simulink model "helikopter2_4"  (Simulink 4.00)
settings: Solver=ode1  SolverMode=SingleTasking  StartTime=0.0  StopTime=999999  FixedStep=0.005  MaxStep=10  RelTol=1e-3  AbsTol=1e-3
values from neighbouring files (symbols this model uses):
  a = [0 0 0;0 0 1;0 0 0]    [init3.m]
  b = [k3 k3;0 0;k1 -k1]    [init3.m]
  c = [ 1 0 0 0 0 0    [init3.m]
  L = (place(a',c',p))'    [init3.m]
undefined symbols (not defined in the file or in its folder): simget
libraries: qctools x7

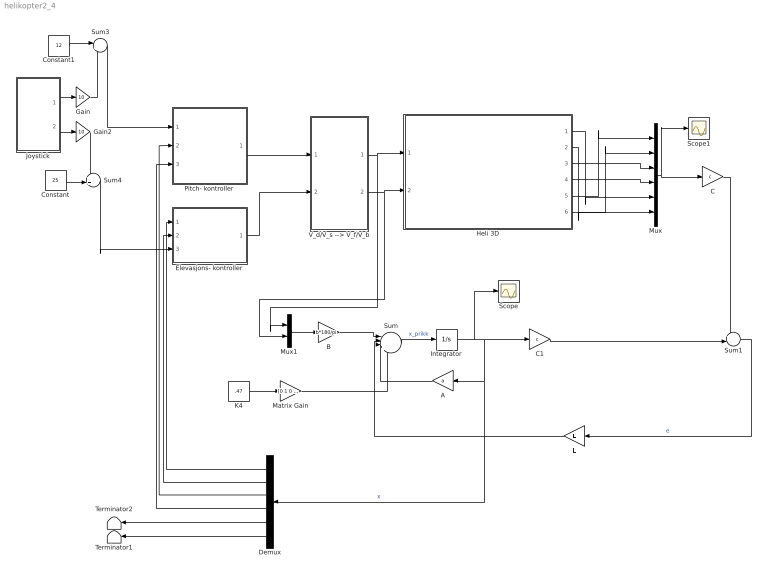
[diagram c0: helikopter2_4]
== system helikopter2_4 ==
  A : Gain  Orientation=left  Gain=a  Multiplication=Matrix(K*u)  SaturateOnIntegerOverflow=on
  B : Gain  Gain=b*180/pi  Multiplication=Matrix(K*u)  SaturateOnIntegerOverflow=on
  C : Gain  Gain=c  Multiplication=Matrix(K*u)  SaturateOnIntegerOverflow=on
  C1 : Gain  Gain=c  Multiplication=Matrix(K*u)  SaturateOnIntegerOverflow=on
  Constant : Constant  Value=25
  Constant1 : Constant  Value=12
  Demux : Demux  Orientation=left  Outputs=6  BusSelectionMode=off
  Elevasjons- kontroller : Subsystem
  Gain : Gain  Gain=10  Multiplication=Element-wise(K.*u)  SaturateOnIntegerOverflow=on
  Gain2 : Gain  Gain=10  Multiplication=Element-wise(K.*u)  SaturateOnIntegerOverflow=on
  Heli 3D : Subsystem
  Integrator : Integrator  ExternalReset=none  InitialConditionSource=internal  InitialCondition=0  LimitOutput=off  UpperSaturationLimit=inf  LowerSaturationLimit=-inf  ShowSaturationPort=off  ShowStatePort=off  AbsoluteTolerance=auto
  Joystick : Subsystem
  K4 : Constant  Value=.47
  L : Gain  Orientation=left  Gain=L  Multiplication=Matrix(K*u)  SaturateOnIntegerOverflow=on
  Matrix Gain : Gain  Gain=[0 1 0 0 0 0]'  Multiplication=Matrix(K*u)  SaturateOnIntegerOverflow=on
  Mux : Mux  Inputs=6
  Mux1 : Mux  Inputs=2
  Pitch- kontroller : Subsystem
  Scope : Scope
  Scope1 : Scope
  Sum : Sum  Inputs=|++++  SaturateOnIntegerOverflow=on
  Sum1 : Sum  Inputs=+-|  SaturateOnIntegerOverflow=on
  Sum3 : Sum  Inputs=|++  SaturateOnIntegerOverflow=on
  Sum4 : Sum  Inputs=++|  SaturateOnIntegerOverflow=on
  Terminator1 : Terminator
  Terminator2 : Terminator
  V_d/V_s --> V_f/V_b : Subsystem
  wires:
  V_d/V_s --> V_f/V_b/2(V_b) -> Heli 3D/2("V_b, motor bak"), Mux1/2
  V_d/V_s --> V_f/V_b/1(V_f) -> Heli 3D/1("V_f, motor foran"), Mux1/1
  Pitch- kontroller/1(V_d) -> V_d/V_s --> V_f/V_b/1(V_d)
  Elevasjons- kontroller/1(V_s) -> V_d/V_s --> V_f/V_b/2(V_s)
  Joystick/1(X Volt) -> Gain/1
  Joystick/2(Y Volt) -> Gain2/1
  Heli 3D/5("Elevasjon, (grader)") -> Mux/1
  Heli 3D/6(Elevasjonsrate (grader/sek)) -> Mux/2
  Heli 3D/3("Pitch, (grader)") -> Mux/3
  Heli 3D/4("Pitchrate, (grader/sek)") -> Mux/4
  Heli 3D/1("Vandring, (grader)") -> Mux/5
  Heli 3D/2("Vandringsrate, (grader/sek)") -> Mux/6
  Gain/1 -> Sum3/2
  B/1 -> Sum/1
  Sum/1 -> Integrator/1  "x_prikk"
  Mux/1 -> C/1, Scope1/1
  Integrator/1 -> C1/1, A/1, Demux/1, Scope/1  "x"
  C1/1 -> Sum1/2
  C/1 -> Sum1/1
  Sum1/1 -> L/1  "e"
  A/1 -> Sum/3
  L/1 -> Sum/2
  Demux/1 -> Elevasjons- kontroller/1("e, grader")
  Demux/2 -> Elevasjons- kontroller/2("e_dot, grader/sek")
  Demux/3 -> Pitch- kontroller/2("p, grader")
  Demux/4 -> Pitch- kontroller/3("p_dot, grader/sek")
  Demux/6 -> Terminator1/1
  Demux/5 -> Terminator2/1
  Constant1/1 -> Sum3/1
  Sum3/1 -> Pitch- kontroller/1("p_c, grader")
  Constant/1 -> Sum4/2
  Gain2/1 -> Sum4/1
  Sum4/1 -> Elevasjons- kontroller/3("e_c, grader")
  Mux1/1 -> B/1
  Matrix Gain/1 -> Sum/4
  K4/1 -> Matrix Gain/1

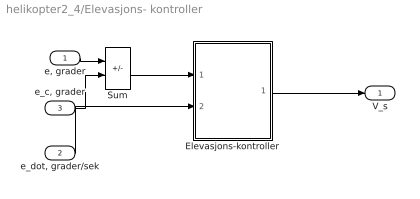
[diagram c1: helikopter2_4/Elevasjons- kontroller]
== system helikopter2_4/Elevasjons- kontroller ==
  "e, grader" : Inport  Port=1  LatchInput=off
  "e_dot, grader/sek" : Inport  Port=2  LatchInput=off
  "e_c, grader" : Inport  Port=3  LatchInput=off
  Elevasjons-kontroller : Subsystem
  Sum : Sum  Inputs=-+  SaturateOnIntegerOverflow=on
  V_s : Outport  Port=1  InitialOutput=0
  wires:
  Sum/1 -> Elevasjons-kontroller/1("e, grader")
  Elevasjons-kontroller/1(out_1) -> V_s/1
  "e, grader"/1 -> Sum/1
  "e_dot, grader/sek"/1 -> Elevasjons-kontroller/2("e, grader/sek")
  "e_c, grader"/1 -> Sum/2

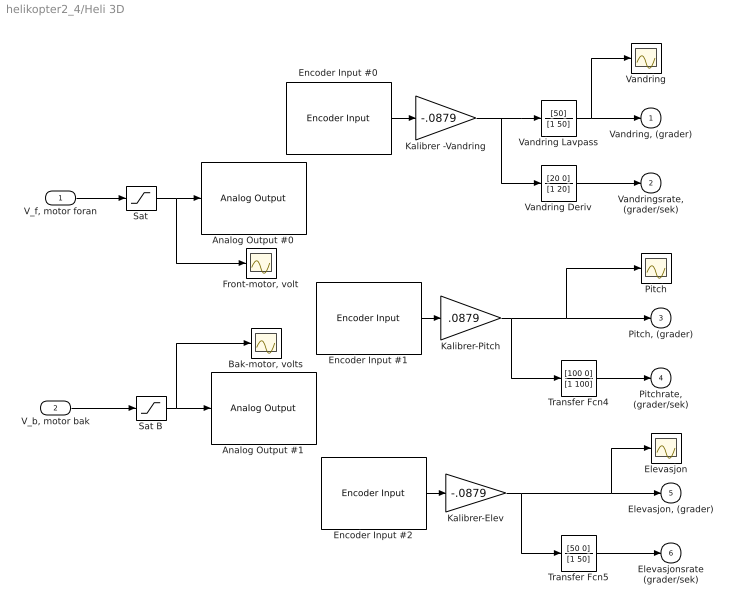
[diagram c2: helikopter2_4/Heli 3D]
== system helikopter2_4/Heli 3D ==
  "V_f, motor foran" : Inport  Port=1  LatchInput=off
  "V_b, motor bak" : Inport  Port=2  LatchInput=off
  Analog Output #0 : qctools/Quanser Consulting MQ3 Series/Analog Output  baseAddr=0x320  channels=0  initialOutputs=0  finalOutputs=0  sampleTime=-1  simulationOutput=off
  Analog Output #1 : qctools/Quanser Consulting MQ3 Series/Analog Output  baseAddr=0x320  channels=1  initialOutputs=0  finalOutputs=0  sampleTime=-1  simulationOutput=off
  "Bak-motor, volts" : Scope
  Elevasjon : Scope
  Encoder Input #0 : qctools/Quanser Consulting MQ3 Series/Encoder Input  baseAddr=0x320  channels=0  initialValues=0  sampleTime=simget(bdroot,'FixedStep')  simulationInput=off
  Encoder Input #1 : qctools/Quanser Consulting MQ3 Series/Encoder Input  baseAddr=0x320  channels=1  initialValues=0  sampleTime=simget(bdroot,'FixedStep')  simulationInput=off
  Encoder Input #2 : qctools/Quanser Consulting MQ3 Series/Encoder Input  baseAddr=0x320  channels=2  initialValues=0  sampleTime=simget(bdroot,'FixedStep')  simulationInput=off
  "Front-motor, volt" : Scope
  Kalibrer -Vandring : Gain  Gain=-.0879  Multiplication=Element-wise(K.*u)  SaturateOnIntegerOverflow=on
  Kalibrer-Elev : Gain  Gain=-.0879  Multiplication=Element-wise(K.*u)  SaturateOnIntegerOverflow=on
  Kalibrer-Pitch : Gain  Gain=.0879  Multiplication=Element-wise(K.*u)  SaturateOnIntegerOverflow=on
  Pitch : Scope
  Sat : Saturate  UpperLimit=5  LowerLimit=-5  LinearizeAsGain=on
  Sat B : Saturate  UpperLimit=5  LowerLimit=-5  LinearizeAsGain=on
  Transfer Fcn4 : TransferFcn  Numerator=[100 0]  Denominator=[1 100]  AbsoluteTolerance=auto  Realization=auto
  Transfer Fcn5 : TransferFcn  Numerator=[50 0]  Denominator=[1 50]  AbsoluteTolerance=auto  Realization=auto
  Vandring : Scope
  Vandring Deriv : TransferFcn  Numerator=[20 0]  Denominator=[1 20]  AbsoluteTolerance=auto  Realization=auto
  Vandring Lavpass : TransferFcn  Numerator=[50]  Denominator=[1 50]  AbsoluteTolerance=auto  Realization=auto
  "Vandring, (grader)" : Outport  Port=1  InitialOutput=0
  "Vandringsrate, (grader/sek)" : Outport  Port=2  InitialOutput=0
  "Pitch, (grader)" : Outport  Port=3  InitialOutput=0
  "Pitchrate, (grader/sek)" : Outport  Port=4  InitialOutput=0
  "Elevasjon, (grader)" : Outport  Port=5  InitialOutput=0
  Elevasjonsrate (grader/sek) : Outport  Port=6  InitialOutput=0
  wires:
  Vandring Deriv/1 -> "Vandringsrate, (grader/sek)"/1
  Vandring Lavpass/1 -> Vandring/1, "Vandring, (grader)"/1
  Encoder Input #0/1 -> Kalibrer -Vandring/1
  Kalibrer -Vandring/1 -> Vandring Deriv/1, Vandring Lavpass/1
  Encoder Input #1/1 -> Kalibrer-Pitch/1
  Kalibrer-Pitch/1 -> Pitch/1, "Pitch, (grader)"/1, Transfer Fcn4/1
  Transfer Fcn4/1 -> "Pitchrate, (grader/sek)"/1
  Encoder Input #2/1 -> Kalibrer-Elev/1
  Kalibrer-Elev/1 -> Transfer Fcn5/1, Elevasjon/1, "Elevasjon, (grader)"/1
  Transfer Fcn5/1 -> Elevasjonsrate (grader/sek)/1
  Sat/1 -> "Front-motor, volt"/1, Analog Output #0/1
  Sat B/1 -> "Bak-motor, volts"/1, Analog Output #1/1
  "V_f, motor foran"/1 -> Sat/1
  "V_b, motor bak"/1 -> Sat B/1

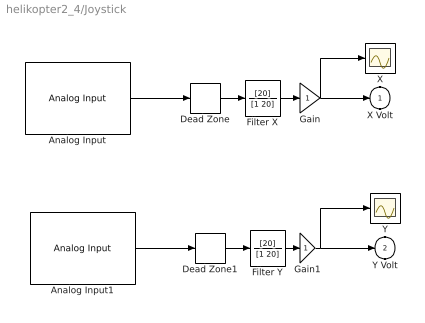
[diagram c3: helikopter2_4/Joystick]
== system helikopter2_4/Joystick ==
  Analog Input : qctools/Quanser Consulting MQ3 Series/Analog Input  baseAddr=0x320  channels=2  sampleTime=simget(bdroot,'FixedStep')  simulationInput=off
  Analog Input1 : qctools/Quanser Consulting MQ3 Series/Analog Input  baseAddr=0x320  channels=3  sampleTime=simget(bdroot,'FixedStep')  simulationInput=off
  Dead Zone : DeadZone  LowerValue=-0.5  UpperValue=0.5  SaturateOnIntegerOverflow=on  LinearizeAsGain=on
  Dead Zone1 : DeadZone  LowerValue=-0.5  UpperValue=0.5  SaturateOnIntegerOverflow=on  LinearizeAsGain=on
  Filter X : TransferFcn  Numerator=[20]  Denominator=[1 20]  AbsoluteTolerance=auto  Realization=auto
  Filter Y : TransferFcn  Numerator=[20]  Denominator=[1 20]  AbsoluteTolerance=auto  Realization=auto
  Gain : Gain  Gain=1  Multiplication=Element-wise(K.*u)  SaturateOnIntegerOverflow=on
  Gain1 : Gain  Gain=1  Multiplication=Element-wise(K.*u)  SaturateOnIntegerOverflow=on
  X : Scope
  Y : Scope
  X Volt : Outport  Port=1  InitialOutput=0
  Y Volt : Outport  Port=2  InitialOutput=0
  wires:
  Dead Zone/1 -> Filter X/1
  Analog Input1/1 -> Dead Zone1/1
  Dead Zone1/1 -> Filter Y/1
  Filter Y/1 -> Gain1/1
  Filter X/1 -> Gain/1
  Analog Input/1 -> Dead Zone/1
  Gain/1 -> X Volt/1, X/1
  Gain1/1 -> Y Volt/1, Y/1

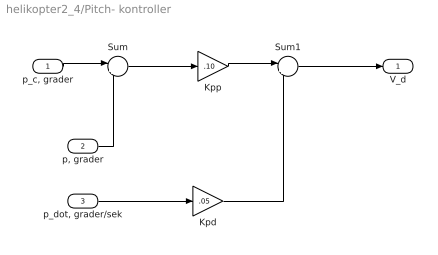
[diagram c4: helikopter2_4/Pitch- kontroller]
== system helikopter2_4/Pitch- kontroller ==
  "p_c, grader" : Inport  Port=1  LatchInput=off
  "p, grader" : Inport  Port=2  LatchInput=off
  "p_dot, grader/sek" : Inport  Port=3  LatchInput=off
  Kpd : Gain  Gain=.05  Multiplication=Element-wise(K.*u)  SaturateOnIntegerOverflow=on
  Kpp : Gain  Gain=.10  Multiplication=Element-wise(K.*u)  SaturateOnIntegerOverflow=on
  Sum : Sum  Inputs=|+-  SaturateOnIntegerOverflow=on
  Sum1 : Sum  Inputs=|+-  SaturateOnIntegerOverflow=on
  V_d : Outport  Port=1  InitialOutput=0
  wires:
  "p_dot, grader/sek"/1 -> Kpd/1
  Sum1/1 -> V_d/1
  Sum/1 -> Kpp/1
  Kpd/1 -> Sum1/2
  "p, grader"/1 -> Sum/2
  "p_c, grader"/1 -> Sum/1
  Kpp/1 -> Sum1/1

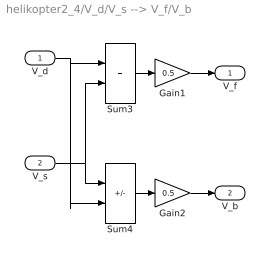
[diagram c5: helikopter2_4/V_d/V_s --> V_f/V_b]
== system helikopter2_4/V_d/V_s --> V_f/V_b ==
  V_d : Inport  Port=1  LatchInput=off
  V_s : Inport  Port=2  LatchInput=off
  Gain1 : Gain  Gain=0.5  Multiplication=Element-wise(K.*u)  SaturateOnIntegerOverflow=on
  Gain2 : Gain  Gain=0.5  Multiplication=Element-wise(K.*u)  SaturateOnIntegerOverflow=on
  Sum3 : Sum  Inputs=++  SaturateOnIntegerOverflow=on
  Sum4 : Sum  Inputs=+-  SaturateOnIntegerOverflow=on
  V_f : Outport  Port=1  InitialOutput=0
  V_b : Outport  Port=2  InitialOutput=0
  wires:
  V_s/1 -> Sum4/1, Sum3/2
  Sum3/1 -> Gain1/1
  Sum4/1 -> Gain2/1
  V_d/1 -> Sum3/1, Sum4/2
  Gain1/1 -> V_f/1
  Gain2/1 -> V_b/1

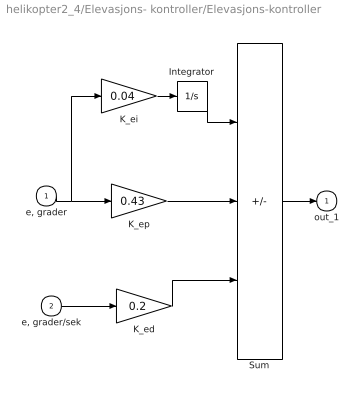
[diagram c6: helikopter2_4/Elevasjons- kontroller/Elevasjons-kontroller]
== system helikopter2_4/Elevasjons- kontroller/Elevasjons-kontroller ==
  "e, grader" : Inport  Port=1  LatchInput=off
  "e, grader/sek" : Inport  Port=2  LatchInput=off
  Integrator : Integrator  ExternalReset=none  InitialConditionSource=internal  InitialCondition=0  LimitOutput=on  UpperSaturationLimit=inf  LowerSaturationLimit=-inf  ShowSaturationPort=off  ShowStatePort=off  AbsoluteTolerance=auto
  K_ed : Gain  Gain=0.2  Multiplication=Element-wise(K.*u)  SaturateOnIntegerOverflow=on
  K_ei : Gain  Gain=0.04  Multiplication=Element-wise(K.*u)  SaturateOnIntegerOverflow=on
  K_ep : Gain  Gain=0.43  Multiplication=Element-wise(K.*u)  SaturateOnIntegerOverflow=on
  Sum : Sum  Inputs=++-  SaturateOnIntegerOverflow=on
  out_1 : Outport  Port=1  InitialOutput=0
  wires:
  K_ei/1 -> Integrator/1
  Integrator/1 -> Sum/1
  Sum/1 -> out_1/1
  "e, grader/sek"/1 -> K_ed/1
  K_ed/1 -> Sum/3
  K_ep/1 -> Sum/2
  "e, grader"/1 -> K_ep/1, K_ei/1
